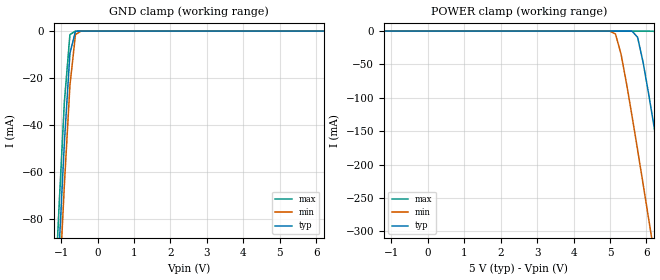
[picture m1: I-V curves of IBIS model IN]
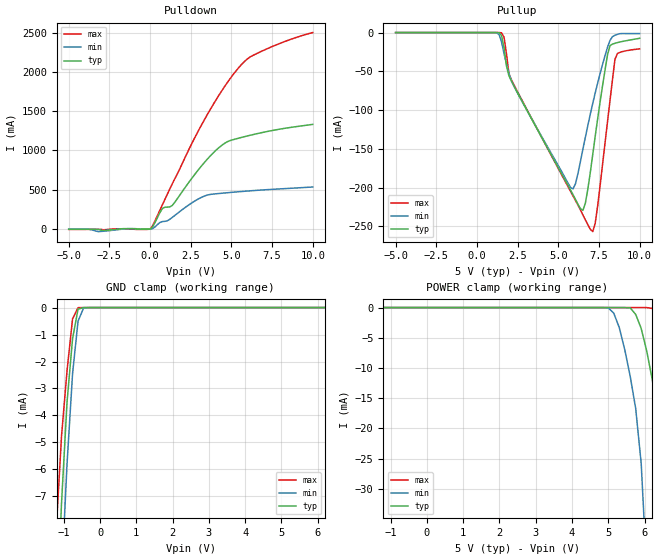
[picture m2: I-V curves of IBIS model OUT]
|   TEXAS INSTRUMENTS INCORPORATED
|   Standard Linear and Logic
|   IBIS Model of SN74ABT16823
|   18-Bit Bus-Interface Flip-Flops with 3-state outputs
|   TSSOP 56-pin (DGG) and SSOP 56-pin (DL) Package
[IBIS Ver]   2.1
[File Name]   sn74abt16823.ibs
[File Rev]   1.1
[Date]   1/4/01
[Source]   File originated at Texas Instruments, Inc.
[Notes]   The following is a sample IBIS file for the ABT16823.
|   - All test data contained in this file are derived from
|   hspice(tm) simulations.
|   - This file may be incomplete or may not be fully compliant
|   with the IBIS specification. It will be replaced with a
|   version that is IBIS Revision 3.2 compliant and is complete
|   and accurate.  Please email all questions and comments to
|   sllibis@ti.com.
|   - File created by Ramzi Ammar, SLL Applications
[Disclaimer] Property of Texas Instruments Incorporated.  Unauthorized
   reproduction and/or distribution is strictly prohibited.
   This product is protected under copyright law.
   Created 1997, (C) Copyright 1997, Texas Instruments Inc.,
   All Rights Reserved
   UNLESS THERE IS A SIGNED, WRITTEN AGREEMENT TO THE
   CONTRARY, TEXAS INSTRUMENTS ("TI") IS PROVIDING THE IBIS
   MODELS "AS IS" AND WITHOUT ANY WARRANTY, EXPRESSED OR
   IMPLIED.  TI assumes no liability for:
   1) the accuracy of the IBIS models provided to your
   company;
   2) the proper functioning of these IBIS models in your
   design or for any resulting applications; or
   3) infringement of patents, copyrights or intellectual
   property rights resulting from your use of these IBIS
   models.
   TI provides IBIS Models as a service to our customers.
   You and your company shall not distribute, sell or give
   these models to anyone else without prior written
   permission from TI.
   TI reserves the right to make changes to our products or
   to discontinue any semiconductor product or service
   without notice, and advises our customers to obtain the
   latest version of relevant information to verify, before
   placing orders, that the information being relied on is
   current.
   Please be aware that your receipt and use of the IBIS
   information provided shall serve as acceptance of these
   terms and conditions.  If you do not accept these terms,
   you should return or destroy the IBIS models and any
   other accompanying information immediately.
[Component]   ABT16823_DGG
[Manufacturer] Texas Instruments.
[Package]
|   typ   min   max
R_pkg   0.045   0.035   0.062
L_pkg   3.324nH   2.403nH   5.094nH
C_pkg   0.564pF   0.341pF   0.914pF
[Pin]   signal_name   model_name   R_pin   L_pin   C_pin
1   1CLR_BAR   NC   0.062   5.094nH   0.856pF
2   1OE_BAR   NC   0.061   4.621nH   0.902pF
3   1Q1   OUT   0.06   4.316nH   0.802pF
4   GND   GND   0.059   3.968nH   0.698pF
5   1Q2   OUT   0.057   3.716nH   0.649pF
6   1Q3   OUT   0.042   3.517nH   0.652pF
7   VCC   POWER   0.041   3.16nH   0.57pF
8   1Q4   OUT   0.039   2.981nH   0.482pF
9   1Q5   OUT   0.039   2.809nH   0.447pF
10   1Q6   OUT   0.038   2.715nH   0.409pF
11   GND   GND   0.041   2.675nH   0.391pF
12   1Q7   OUT   0.039   2.536nH   0.366pF
13   1Q8   OUT   0.039   2.457nH   0.348pF
14   1Q9   OUT   0.038   2.411nH   0.353pF
15   2Q10   OUT   0.039   2.456nH   0.355pF
16   2Q2   OUT   0.039   2.471nH   0.349pF
17   2Q3   OUT   0.04   2.58nH   0.37pF
18   GND   GND   0.038   2.651nH   0.389pF
19   2Q4   OUT   0.038   2.739nH   0.411pF
20   2Q5   OUT   0.039   2.838nH   0.449pF
21   2Q6   OUT   0.038   2.988nH   0.484pF
22   VCC   POWER   0.038   3.105nH   0.564pF
23   2Q7   OUT   0.04   3.427nH   0.638pF
24   2Q8   OUT   0.056   3.654nH   0.641pF
25   GND   GND   0.057   3.932nH   0.7pF
26   2Q9   OUT   0.058   4.257nH   0.806pF
27   2OE_BAR   NC   0.057   4.58nH   0.914pF
28   2CLR_BAR   NC   0.059   5.038nH   0.861pF
29   2CLK   NC   0.06   5.058nH   0.858pF
30   2CLKEN_BAR   NC   0.056   4.543nH   0.904pF
31   2D9   IN   0.057   4.24nH   0.803pF
32   GND   GND   0.057   3.929nH   0.7pF
33   2D8   IN   0.056   3.616nH   0.637pF
34   2D7   IN   0.037   3.368nH   0.64pF
35   VCC   POWER   0.036   3.024nH   0.563pF
36   2D6   IN   0.035   2.876nH   0.474pF
37   2D5   IN   0.035   2.745nH   0.444pF
38   2D4   IN   0.037   2.683nH   0.405pF
39   GND   GND   0.038   2.603nH   0.382pF
40   2D3   IN   0.038   2.51nH   0.362pF
41   2D2   IN   0.036   2.412nH   0.341pF
42   2D1   IN   0.038   2.416nH   0.349pF
43   1D9   IN   0.037   2.403nH   0.349pF
44   1D8   IN   0.037   2.429nH   0.341pF
45   1D7   IN   0.036   2.482nH   0.358pF
46   GND   GND   0.037   2.615nH   0.381pF
47   1D6   IN   0.035   2.669nH   0.402pF
48   1D5   IN   0.036   2.763nH   0.442pF
49   1D4   IN   0.036   2.942nH   0.478pF
50   VCC   POWER   0.035   3.053nH   0.564pF
51   1D3   IN   0.036   3.409nH   0.641pF
52   1D2   IN   0.058   3.698nH   0.641pF
53   GND   GND   0.059   3.975nH   0.697pF
54   1D1   IN   0.061   4.327nH   0.802pF
55   1CLKEN_BAR   NC   0.061   4.624nH   0.905pF
56   1CLK   NC   0.06   5.063nH   0.858pF
[Component]   ABT16823_DL
[Manufacturer] Texas Instruments.
[Package]
|   typ   min   max
R_pkg   0.055   0.048   0.067
L_pkg   6.539nH   4.802nH   9.746nH
C_pkg   0.188pF   0.076pF   0.517pF
[Pin]   signal_name   model_name   R_pin   L_pin   C_pin
1   1CLR_BAR   NC   0.064   9.646nH   0.513pF
2   1OE_BAR   NC   0.059   8.723nH   0.27pF
3   1Q1   OUT   0.059   8.139nH   0.223pF
4   GND   GND   0.056   7.554nH   0.201pF
5   1Q2   OUT   0.054   6.991nH   0.195pF
6   1Q3   OUT   0.053   6.659nH   0.202pF
7   VCC   POWER   0.055   6.321nH   0.207pF
8   1Q4   OUT   0.055   5.942nH   0.133pF
9   1Q5   OUT   0.057   5.767nH   0.132pF
10   1Q6   OUT   0.054   5.459nH   0.121pF
11   GND   GND   0.051   5.224nH   0.14pF
12   1Q7   OUT   0.048   5.088nH   0.126pF
13   1Q8   OUT   0.05   5.021nH   0.096pF
14   1Q9   OUT   0.051   4.802nH   0.076pF
15   2Q10   OUT   0.051   4.803nH   0.076pF
16   2Q2   OUT   0.05   5.021nH   0.096pF
17   2Q3   OUT   0.048   5.088nH   0.126pF
18   GND   GND   0.051   5.224nH   0.14pF
19   2Q4   OUT   0.054   5.459nH   0.121pF
20   2Q5   OUT   0.057   5.768nH   0.133pF
21   2Q6   OUT   0.055   5.942nH   0.133pF
22   VCC   POWER   0.055   6.32nH   0.206pF
23   2Q7   OUT   0.053   6.659nH   0.203pF
24   2Q8   OUT   0.054   6.991nH   0.196pF
25   GND   GND   0.056   7.554nH   0.201pF
26   2Q9   OUT   0.059   8.139nH   0.223pF
27   2OE_BAR   NC   0.059   8.727nH   0.27pF
28   2CLR_BAR   NC   0.067   9.746nH   0.517pF
29   2CLK   NC   0.063   9.63nH   0.511pF
30   2CLKEN_BAR   NC   0.06   8.751nH   0.271pF
31   2D9   IN   0.06   8.184nH   0.225pF
32   GND   GND   0.056   7.543nH   0.2pF
33   2D8   IN   0.054   7.005nH   0.196pF
34   2D7   IN   0.056   6.714nH   0.204pF
35   VCC   POWER   0.058   6.384nH   0.208pF
36   2D6   IN   0.057   5.976nH   0.134pF
37   2D5   IN   0.057   5.743nH   0.13pF
38   2D4   IN   0.054   5.468nH   0.119pF
39   GND   GND   0.055   5.328nH   0.142pF
40   2D3   IN   0.052   5.189nH   0.129pF
41   2D2   IN   0.052   5.053nH   0.096pF
42   2D1   IN   0.051   4.825nH   0.076pF
43   1D9   IN   0.054   4.896nH   0.078pF
44   1D8   IN   0.052   5.093nH   0.097pF
45   1D7   IN   0.051   5.179nH   0.128pF
46   GND   GND   0.054   5.314nH   0.142pF
47   1D6   IN   0.055   5.511nH   0.121pF
48   1D5   IN   0.057   5.771nH   0.131pF
49   1D4   IN   0.056   5.957nH   0.133pF
50   VCC   POWER   0.055   6.32nH   0.206pF
51   1D3   IN   0.052   6.621nH   0.2pF
52   1D2   IN   0.053   6.973nH   0.195pF
53   GND   GND   0.057   7.571nH   0.202pF
54   1D1   IN   0.057   8.097nH   0.222pF
55   1CLKEN_BAR   NC   0.059   8.723nH   0.271pF
56   1CLK   NC   0.061   9.56nH   0.509pF
| Models and submodels in the file (2): IN (Input), OUT (Output)
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|   Model ABT16823_IN
[Model]   IN
Model_type  Input
Polarity   Non-Inverting
Vinl = 0.8
Vinh = 2.0
| variable   typ   min   max
C_comp   3.5p   NA   NA
[Temperature Range]   50   0   100
[Voltage range]   5.0   4.5   5.5
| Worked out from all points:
|   GND clamp passes 1 mA (typ) near -0.62 V on its own axis
[gnd_clamp]
|   50C:5V:   100C:4.5V:weak   0C:5.5V:strong
|   Voltage   I(typ)   I(min)   I(max)
-5V       -1.478A    -1.495A    -1.463A
-1.212V   -144.4mA   -163mA     -126.1mA
-1.061V   -94.48mA   -113mA     -76.16mA
-909.5mV  -47.26mA   -65.22mA   -29.93mA
-758mV    -9.437mA   -23.15mA   -1.506mA
-606.5mV  -118.2uA   -1.475mA   -3.365uA
-455mV    -587.2nA   -17.09uA   -6.307nA
9.998V    2nA        2.016nA    2nA
[power_clamp]
|   50C:5V:   100C:4.5V:weak   0C:5.5V:strong
|   Voltage   I(typ)   I(min)   I(max)
-5V       2nA        1.917nA    2.1nA
4.999V    202.3fA    -64.74uA   100.2pA
5.151V    -43.34pA   -4.362mA   69.9pA
5.302V    -2.783nA   -34.28mA   39.6pA
5.756V    -9.181mA   -177.7mA   -52.93pA
6.059V    -93.99mA   -280.9mA   -477.7nA
6.211V    -143.9mA   -333.2mA   -249.7uA
6.362V    -195.1mA   -385.8mA   -17.65mA
6.665V    -299.3mA   -491.6mA   -110.4mA
7.12V     -457.9mA   -651.2mA   -265.7mA
7.271V    -511.1mA   -704.5mA   -318.4mA
9.998V    -1.478A    -1.672A    -1.284A
|   Model ABT16823_OUT
[Model]   OUT
Model_type  Output
Polarity   Non-Inverting
Enable   Active-Low
Vinl = 0.8
Vinh = 2.0
| variable   typ   min   max
C_comp   7.5p   NA   NA
[Temperature Range]   50   0   100
[Voltage range]   5.0   4.5   5.5
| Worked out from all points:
|   slope of the pulldown table from 0 to 0.75 V, typ, clamps not added: 2.9 ohm
|   GND clamp passes 1 mA (typ) near -0.74 V on its own axis
[pullup]
|   50C:5V:   100C:4.5V:weak   0C:5.5V:strong
|   Voltage   I(typ)   I(min)   I(max)
-5V       307.6pA    513.3pA    117.5pA
1.212V    -24.3uA    -309.9uA   -650.2nA
1.514V    -4.019mA   -12.23mA   -390.1uA
2.12V     -62.55mA   -62.17mA   -60.93mA
5.756V    -203mA     -199.8mA   -204.8mA
6.059V    -215.3mA   -194.8mA   -216.6mA
6.514V    -229.3mA   -150.4mA   -235.2mA
7.12V     -157mA     -91.21mA   -256.7mA
7.423V    -110.8mA   -64.9mA    -223.1mA
8.029V    -28.43mA   -18.82mA   -114.5mA
8.483V    -13.85mA   -3.493mA   -34.49mA
9.998V    -7.413mA   -1.335mA   -21.02mA
[pulldown]
|   50C:5V:   100C:4.5V:weak   0C:5.5V:strong
|   Voltage   I(typ)   I(min)   I(max)
-5V       -4.326mA   -1.526mA   -8.46mA
-3.182V   -6.391mA   -35.75mA   -6.209mA
-500uV    -2.416mA   -1.496mA   -3.964mA
151mV     22.83mA    1.569mA    37.87mA
757mV     259.1mA    92.62mA    306.2mA
1.363V    297.3mA    145.1mA    573.1mA
2.878V    728.3mA    370.5mA    1.213A
3.787V    947.1mA    440.9mA    1.552A
4.545V    1.084A     456.1mA    1.802A
5.302V    1.147A     470.1mA    2.017A
6.362V    1.202A     487.4mA    2.213A
9.998V    1.331A     532.9mA    2.501A
[gnd_clamp]
|   50C:5V:   100C:4.5V:weak   0C:5.5V:strong
|   Voltage   I(typ)   I(min)   I(max)
-5V       -573.2mA   -564.7mA   -581.9mA
-1.212V   -11.93mA   -15.01mA   -8.344mA
-1.061V   -7.224mA   -10.04mA   -4.745mA
-909.5mV  -3.495mA   -5.785mA   -2.333mA
-758mV    -1.153mA   -2.451mA   -419.8uA
-606.5mV  -57.4uA    -502.1uA   -3.912uA
-455mV    -590.2nA   -18.57uA   -111.6nA
-303.5mV  -56.81nA   -424.5nA   -77.78nA
9.998V    5.955nA    6.238nA    5.684nA
[power_clamp]
|   50C:5V:   100C:4.5V:weak   0C:5.5V:strong
|   Voltage   I(typ)   I(min)   I(max)
-5V       5.956nA    5.926nA    5.916nA
4.999V    -6.903nA   -52.88uA   246.2pA
5.302V    -56.47nA   -3.29mA    62.69pA
5.756V    -1.135mA   -16.73mA   -74.71nA
6.059V    -7.181mA   -43.67mA   -855nA
6.211V    -11.88mA   -68.42mA   -133.5uA
6.362V    -17.41mA   -96.1mA    -1.654mA
6.665V    -47.98mA   -153.6mA   -6.989mA
6.968V    -111.8mA   -210.6mA   -17.98mA
7.12V     -147.2mA   -238.5mA   -27.35mA
7.271V    -183.2mA   -266.1mA   -51.03mA
9.998V    -573mA     -618.6mA   -529.2mA
[ramp]
| variable   typ   min   max
dV/dt_r   1.8548E+00/1.2707E-09  1.6037E+00/6.7257E-10  2.0195E+00/1.1847E-09
dV/dt_f   2.7994E+00/1.1353E-09  2.3525E+00/1.3259E-09  3.1148E+00/8.5697E-10
